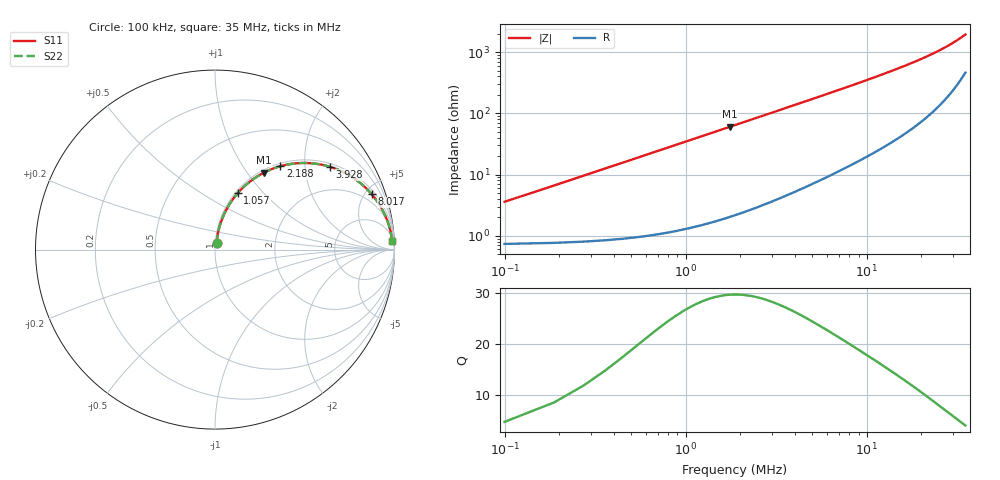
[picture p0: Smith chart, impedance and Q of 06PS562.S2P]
! Coilcraft 0603PS-562 Power Chip Inductor
! 19 February 2003
# MHZ S MA R 50
!Freq  MagS11  AngS11  MagS21  AngS21  MagS12  AngS12  MagS22  AngS22
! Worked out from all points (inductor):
!   403 points, 100 kHz to 35 MHz, reference 50 ohm
!   read as one part in series: L = 5.54 uH near 274 kHz
!   highest Q = 29.6 at 1.753 MHz (marker M1), where L = 5.46 uH
!   S11 on the Smith chart (normalised r, x): 100 kHz: 1.01, +0.07; 1.057 MHz: 1.03, +0.73; 2.188 MHz: 1.05, +1.50; 3.928 MHz: 1.10, +2.69; 8.017 MHz: 1.28, +5.54; 35 MHz: 10, +38
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0.1  0.03565 76.2  0.9921 -2.0  0.9921 -2.0  0.03565 76.2
0.187  0.06523 79.6  0.9903 -3.7  0.9903 -3.7  0.06523 79.6
0.361  0.1238 79.1  0.984 -7.1  0.984 -7.1  0.1238 79.1
0.448  0.1526 78.0  0.9796 -8.8  0.9796 -8.8  0.1526 78.0
0.535  0.1809 76.7  0.9743 -10.4  0.9743 -10.4  0.1809 76.7
0.622  0.2087 75.3  0.9683 -12.0  0.9683 -12.0  0.2087 75.3
0.796  0.2626 72.4  0.9542 -15.2  0.9542 -15.2  0.2626 72.4
1.057  0.3385 68.1  0.9286 -19.8  0.9286 -19.8  0.3385 68.1
1.405  0.4294 62.6  0.8885 -25.4  0.8885 -25.4  0.4294 62.6
1.753  0.5083 57.5  0.8443 -30.5  0.8443 -30.5  0.5083 57.5
2.188  0.5906 51.9  0.7872 -36.2  0.7872 -36.2  0.5906 51.9
3.058  0.7107 42.7  0.6788 -45.3  0.6788 -45.3  0.7107 42.7
3.928  0.7882 35.9  0.5863 -52.0  0.5863 -52.0  0.7882 35.9
4.885  0.8435 30.2  0.504 -57.4  0.504 -57.4  0.8435 30.2
5.929  0.8824 25.7  0.4336 -61.8  0.4336 -61.8  0.8824 25.7
8.017  0.926 19.5  0.3341 -67.6  0.3341 -67.6  0.926 19.5
9.67  0.9447 16.2  0.2802 -70.6  0.2802 -70.6  0.9447 16.2
11.758  0.9589 13.3  0.2307 -73.2  0.2307 -73.2  0.9589 13.3
17.587  0.9767 8.5  0.1482 -76.7  0.1482 -76.7  0.9767 8.5
23.416  0.9832 5.8  0.1024 -77.6  0.1024 -77.6  0.9832 5.8
29.245  0.9858 4.1  0.07231 -76.7  0.07231 -76.7  0.9858 4.1
35  0.9867 2.8  0.0508 -73.4  0.0508 -73.4  0.9867 2.8
